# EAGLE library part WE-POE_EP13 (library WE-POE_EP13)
Transformer for Power-over-Ethernet WE-PoE - Flyback converter transducer particularly for PoE PDs - Insulation voltage 1,5 kVAC/1 min - Input voltages 36V till 57V -- Flyback converters -- Power-over-Ethernet PDs
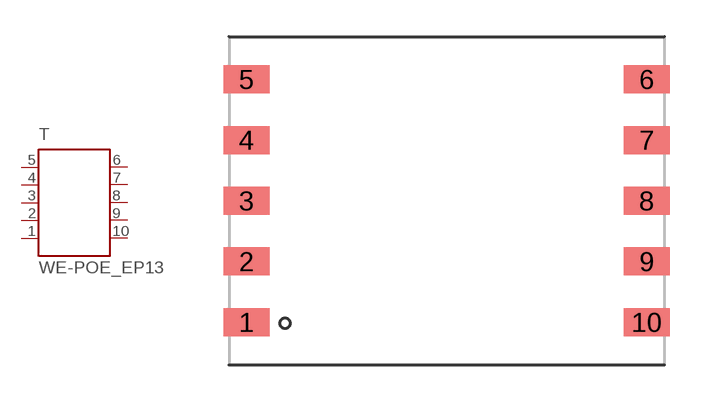
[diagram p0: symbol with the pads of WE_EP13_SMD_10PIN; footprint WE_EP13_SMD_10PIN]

Designator prefix T

## WE-POE_EP13, WE-POE_EP13-7491199112 (MPN: 7491199112; OC_FARNELL: 1849012; OC_NEWARK: 13T9817; PACKAGE: EP13; SUPPLIER: Wuerth Elektronik), WE-POE_EP13-7491199212 (MPN: 7491199212; OC_FARNELL: 1849014; OC_NEWARK: 13T9818; PACKAGE: EP13; SUPPLIER: Wuerth Elektronik), WE-POE_EP13-7491199312 (MPN: 7491199312; OC_FARNELL: 1849017; OC_NEWARK: 13T9819; PACKAGE: EP13; SUPPLIER: Wuerth Elektronik), WE-POE_EP13-749119933 (MPN: 749119933; OC_FARNELL: 1849008; OC_NEWARK: 13T9820; PACKAGE: EP13; SUPPLIER: Wuerth Elektronik), WE-POE_EP13-7491199331 (MPN: 7491199331; OC_FARNELL: 1849009; OC_NEWARK: 13T9821; PACKAGE: EP13; SUPPLIER: Wuerth Elektronik), WE-POE_EP13-7491199332 (MPN: 7491199332; OC_FARNELL: 1849016; OC_NEWARK: 13T9822; PACKAGE: EP13; SUPPLIER: Wuerth Elektronik), WE-POE_EP13-749119950 (MPN: 749119950; OC_FARNELL: 1849010; OC_NEWARK: 13T9823; PACKAGE: EP13; SUPPLIER: Wuerth Elektronik), WE-POE_EP13-7491199501 (MPN: 7491199501; OC_FARNELL: 1849011; OC_NEWARK: 13T9824; PACKAGE: EP13; SUPPLIER: Wuerth Elektronik), WE-POE_EP13-750310013 (MPN: 750310013; OC_FARNELL: 1849015; OC_NEWARK: 13T9825; PACKAGE: EP13; SUPPLIER: Wuerth Elektronik)  [WE_EP13_SMD_10PIN]
1  5  pas
2  4  pas
3  3  pas
4  2  pas
5  1  pas
6  10  pas
7  9  pas
8  8  pas
9  7  pas
10  6  pas

## Footprint WE_EP13_SMD_10PIN (pad centres in mm)
Transformer, EP13 SMD 10 Pin
smd 1.88 x 1.143: 1 -8.18,-4.96; 2 -8.18,-2.48; 3 -8.18,0; 4 -8.18,2.48; 5 -8.18,4.96; 6 8.18,4.96; 7 8.18,2.48; 8 8.18,0; 9 8.18,-2.48; 10 8.18,-4.96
